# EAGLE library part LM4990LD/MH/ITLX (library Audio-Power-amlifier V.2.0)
The LM4990 is an audio power amplifier primarily designed for demanding applications in mobile phones and other portable communication device applications. It is capable of delivering 1.25 watts of continuous average power to an 8Ω BTL load and 2 watts of continuous average power (LD and MH only) to a 4Ω BTL load with less than 1% distortion (THD+N+N) from a 5VDC power supply.
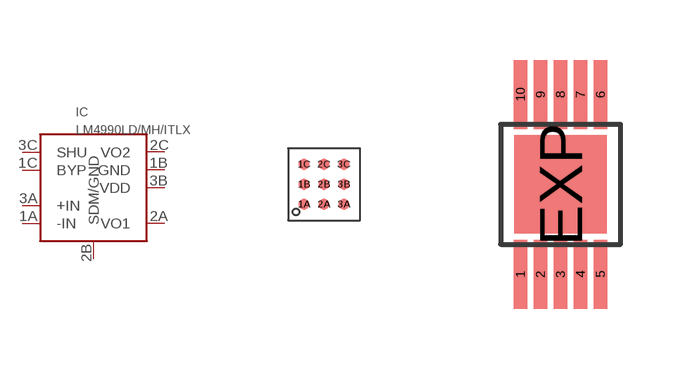
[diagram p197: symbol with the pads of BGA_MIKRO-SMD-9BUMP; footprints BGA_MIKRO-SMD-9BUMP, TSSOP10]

Designator prefix IC

## LM4990LD/MH/ITLXLM4990ITLX  [BGA_MIKRO-SMD-9BUMP]
1A  -IN  in
1B  GND  pwr
1C  BYP
2A  VO1  out
2B  SDM/GND
2C  VO2  out
3A  +IN  in
3B  VDD  pwr
3C  SHU

## LM4990LD/MH/ITLXLM4990MH  [TSSOP10]
1  SHU
2  BYP
3  SDM/GND
4  +IN  in
5  -IN  in
6  VO1  out
8  VDD  pwr
9  GND  pwr
10  VO2  out

## LM4990LD/MH/ITLXLM4990LD  [LLP10-LDA10B]
Pads as for TSSOP10

## Footprint BGA_MIKRO-SMD-9BUMP (pad centres in mm)
BGA-Package Number TLA09 www.national.com
smd 0.277 x 0.277: 1A -0.5,-0.5; 1B -0.5,0; 1C -0.5,0.5; 2A 0,-0.5; 2B 0,0; 2C 0,0.5; 3A 0.5,-0.5; 3B 0.5,0; 3C 0.5,0.5

## Footprint TSSOP10 (pad centres in mm)
TSSOP10 Package Number MXF10A. www.national.com
smd 0.33 x 1.73: 1 -1,-2.25; 2 -0.5,-2.25; 3 0,-2.25; 4 0.5,-2.25; 5 1,-2.25; 6 1,2.25; 7 0.5,2.25; 8 0,2.25; 9 -0.5,2.25; 10 -1,2.25
smd 2.32 x 2.46: EXP 0,0

## Footprint LLP10-LDA10B (pad centres in mm)
LLP10 -Package Number LDA10B 3x4 body. www.national.com
smd 0.26 x 0.51: 1 1,1.65; 2 0.5,1.65; 3 0,1.65; 4 -0.5,1.65; 5 -1,1.65; 6 -1,-1.65; 7 -0.5,-1.65; 8 0,-1.65; 9 0.5,-1.65; 10 1,-1.65
smd 2 x 2.2: EXP 0,0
